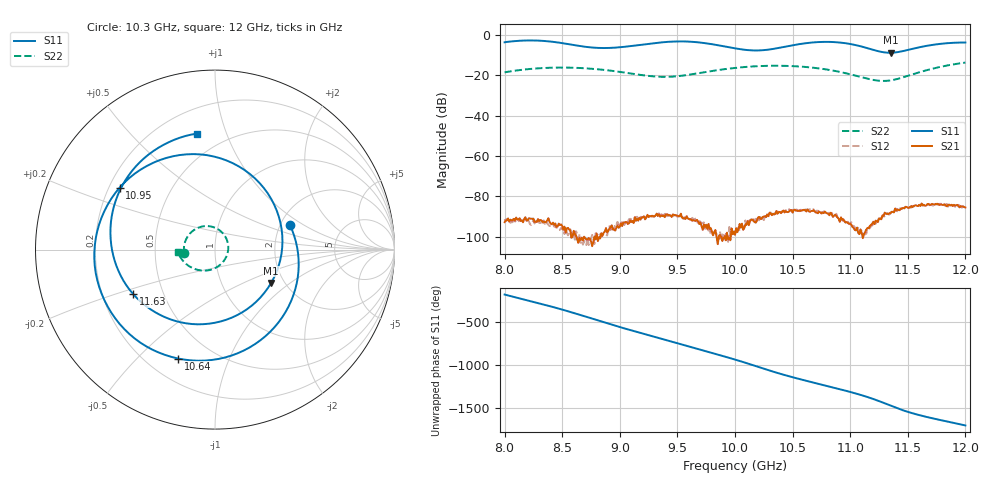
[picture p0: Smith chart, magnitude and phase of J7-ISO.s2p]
!Keysight Technologies,N5234A,MY52241180,A.10.60.03
!Date: Tuesday, May 30, 2023 15:26:06
!Correction: S11(Full 2 Port(1,2))
!S21(Full 2 Port(1,2))
!S12(Full 2 Port(1,2))
!S22(Full 2 Port(1,2))
!S2P File: Measurements: S11, S21, S12, S22:
# Hz S  dB  R 50
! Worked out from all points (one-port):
!   401 points, 8 GHz to 12 GHz, reference 50 ohm
!   lowest |S11| = -8.8 dB at 11.35 GHz (marker M1), VSWR 2.14, Z = 85.7 - j36.6 ohm
!   |S11| at or under -10 dB: nowhere
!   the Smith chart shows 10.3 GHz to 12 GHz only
!   S11 on the Smith chart (normalised r, x): 10.3 GHz: 2.25, +0.77; 10.64 GHz: 0.32, -0.67; 10.95 GHz: 0.24, +0.28; 11.63 GHz: 0.34, -0.23; 12 GHz: 0.35, +0.80
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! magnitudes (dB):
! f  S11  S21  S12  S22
! 8 GHz  -3.6  -92.8  -91.3  -18.5
! 8.15 GHz  -2.8  -92.0  -91.7  -17.2
! 8.3 GHz  -2.8  -92.3  -93.1  -16.5
! 8.67 GHz  -5.6  -100.5  -102.2  -16.4
! 8.92 GHz  -6.4  -95.4  -96.8  -17.6
! 9.34 GHz  -3.8  -88.9  -88.5  -20.7
! 9.48 GHz  -3.2  -89.4  -89.3  -20.5
! 9.64 GHz  -3.4  -91.8  -91.7  -19.3
! 10 GHz  -6.6  -99.0  -99.0  -16.3
! 10.16 GHz  -7.6  -92.1  -91.3  -15.5
! 10.3 GHz  -7.1  -88.1  -88.4  -15.2
! 10.64 GHz  -3.9  -87.4  -86.6  -16.0
! 10.67 GHz  -3.7  -87.2  -86.9  -16.1
! 10.82 GHz  -3.4  -89.4  -88.9  -17.3
! 10.95 GHz  -4.0  -92.2  -92.3  -18.8
! 11.21 GHz  -7.5  -93.8  -92.8  -22.3
! 11.34 GHz  -8.8  -88.4  -89.0  -22.6
! 11.35 GHz  -8.8  -88.5  -88.0  -22.5
! 11.43 GHz  -8.3  -86.9  -86.0  -21.5
! 11.63 GHz  -5.7  -84.6  -84.0  -18.0
! 11.81 GHz  -4.2  -84.2  -84.1  -15.4
! 12 GHz  -3.7  -85.5  -84.8  -13.6
